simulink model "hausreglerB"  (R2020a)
settings: Solver=ode45  StartTime=0.0  StopTime=400  MaxStep=1  RelTol=1e-3  EnableMultiTasking=on
libraries: libregler1B x2

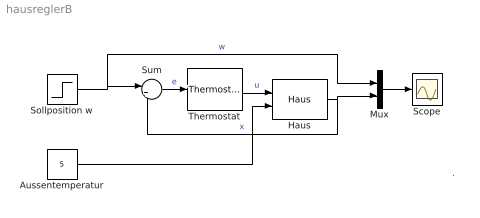
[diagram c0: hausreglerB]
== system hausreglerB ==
  note: .
  Aussentemperatur : Constant  Value=5
  Haus : libregler1B/Haus  C=100000  R=0.001  T0=16
  Mux : Mux  Inputs=2
  Scope : Scope
  Sollposition w : Step  After=20  SampleTime=0
  Sum : Sum  Inputs=|+-  SaturateOnIntegerOverflow=on
  Thermostat : libregler1B/Thermostat  umax=18500  delta=0.5
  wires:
  Thermostat/1 -> Haus/1  "u"
  Haus/1 -> Sum/2, Mux/2  "x"
  Sollposition w/1 -> Sum/1, Mux/1  "w"
  Sum/1 -> Thermostat/1  "e"
  Mux/1 -> Scope/1
  Aussentemperatur/1 -> Haus/2
